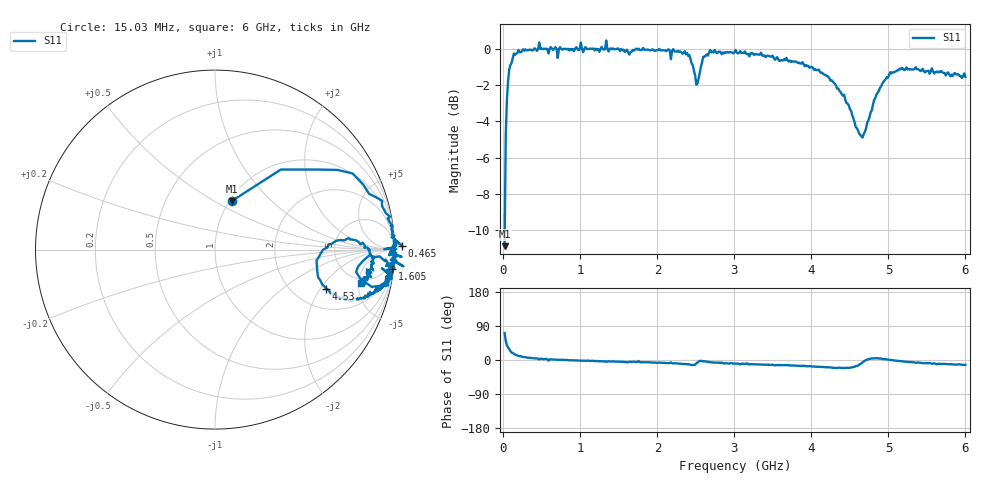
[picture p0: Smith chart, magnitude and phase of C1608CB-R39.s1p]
!	Network	Analyzer	HP8753E.07.74:	Oct	30	2002	Serial	No.	JP38451487
!	Hewlett-Packard
!	27	Aug	2009	14:32:52
!	Frequency	S11
#	HZ	S	RI	R	50
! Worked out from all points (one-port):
!   400 points, 15.03 MHz to 6 GHz, reference 50 ohm
!   lowest |S11| = -10.9 dB at 15.03 MHz (marker M1), VSWR 1.80, Z = 51.2 + j30.1 ohm
!   |S11| at or under -10 dB: start of sweep to 17.21 MHz
!   S11 on the Smith chart (normalised r, x): 15.03 MHz: 1.02, +0.60; 465 MHz: -39, +21; 1.605 GHz: 1, -18; 4.53 GHz: 2.95, -2.26; 6 GHz: 4.38, -5.43
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1.502992e7  0.0925 0.27
3.002985e7  0.367 0.446
6.00297e7  0.683 0.444
1.350293e8  0.931 0.272
4.650277e8  1.04 0.0227
7.050265e8  0.943 0.00259
7.650262e8  0.994 0.0152
1.245024e9  0.979 -0.0591
1.335023e9  1.05 -0.093
1.515022e9  0.982 -0.0775
1.605022e9  0.988 -0.11
1.755021e9  1 -0.043
1.785021e9  0.986 -0.11
2.265019e9  0.974 -0.154
2.415018e9  0.942 -0.188
2.505017e9  0.786 -0.125
2.550017e9  0.86 -0.0316
2.685017e9  0.987 -0.101
3.015015e9  0.978 -0.166
3.765011e9  0.894 -0.224
4.275009e9  0.761 -0.287
4.515007e9  0.635 -0.227
4.530007e9  0.619 -0.218
4.665007e9  0.566 -0.0611
4.845006e9  0.745 0.0641
5.025005e9  0.862 -0.00226
5.265004e9  0.876 -0.084
6e9  0.816 -0.186
